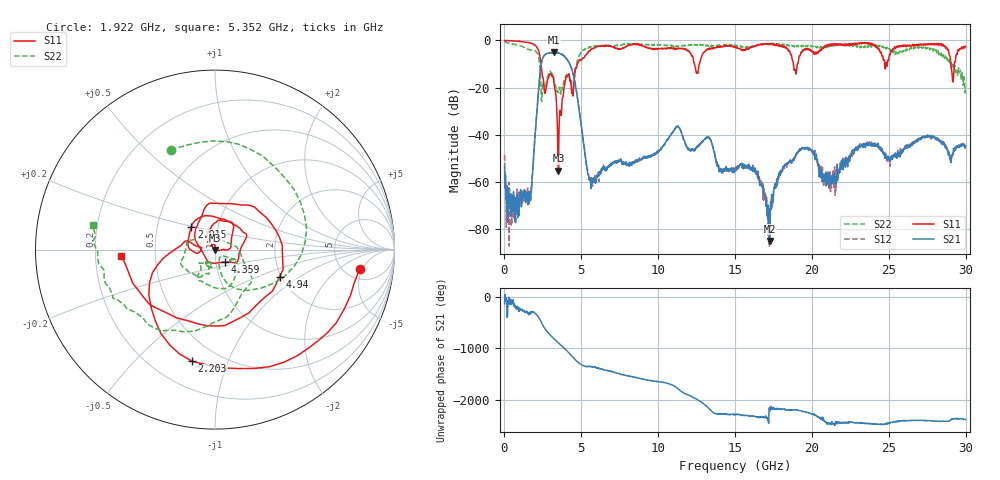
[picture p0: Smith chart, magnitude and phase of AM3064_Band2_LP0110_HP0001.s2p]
# Hz S DB R 50.0
!freq dBS11 angS11 dBS21 angS21 dBS12 angS12 dBS22 angS22
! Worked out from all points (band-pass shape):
!   1600 points, 10 MHz to 29.98 GHz, reference 50 ohm
!   highest |S21| = -5.00 dB at 3.234 GHz (marker M1); lowest = -84.9 dB at 17.27 GHz (marker M2)
!   |S21| within 3 dB of the highest: 2.462 GHz to 4.067 GHz (1.605 GHz wide, 49.2 % of centre)
!   lowest |S11| = -55.2 dB at 3.515 GHz (marker M3), VSWR 1.00, Z = 49.9 - j0.162 ohm
!   |S11| at or under -10 dB: 2.377 GHz to 4.741 GHz (2.364 GHz wide, 66.4 % of centre); 12.36 GHz to 12.67 GHz (317 MHz wide, 2.53 % of centre); 18.8 GHz to 19.05 GHz (253.7 MHz wide, 1.34 % of centre)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
!   |S22| runs from -25.8 to -0.2 dB; largest |S21 - S12| = 0.024
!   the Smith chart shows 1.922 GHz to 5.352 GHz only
!   S11 on the Smith chart (normalised r, x): 1.922 GHz: 6.80, -4.40; 2.203 GHz: 0.36, -0.75; 2.915 GHz: 0.74, +0.19; 4.359 GHz: 1.11, -0.15; 4.94 GHz: 1.96, -0.70; 5.352 GHz: 0.31, -0.03
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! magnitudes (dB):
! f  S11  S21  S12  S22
! 10 MHz  0.0  -53.6  -48.5  -0.2
! 591.1 MHz  -0.2  -64.1  -71.0  -1.6
! 1.622 GHz  -1.0  -66.6  -65.5  -4.0
! 1.922 GHz  -1.8  -46.8  -46.7  -4.3
! 2.203 GHz  -3.9  -22.2  -22.2  -6.3
! 2.522 GHz  -16.3  -7.1  -7.1  -17.4
! 2.915 GHz  -14.8  -5.3  -5.3  -13.4
! 3.234 GHz  -18.7  -5.0  -5.2  -18.0
! 3.515 GHz  -55.2  -5.3  -5.3  -21.9
! 4.359 GHz  -21.0  -11.7  -11.7  -20.0
! 4.94 GHz  -8.2  -33.2  -33.2  -5.3
! 5.015 GHz  -8.3  -36.7  -36.8  -5.1
! 5.352 GHz  -5.6  -53.2  -53.0  -3.2
! 10 GHz  -3.5  -47.0  -47.2  -1.9
! 11.27 GHz  -3.5  -36.5  -36.3  -2.6
! 15 GHz  -2.7  -55.0  -55.1  -2.1
! 17.27 GHz  -1.4  -84.9  -73.8  -1.3
! 18.25 GHz  -3.2  -53.0  -53.0  -1.8
! 19.99 GHz  -4.4  -46.6  -47.3  -2.3
! 21.25 GHz  -1.5  -59.0  -59.6  -2.5
! 25 GHz  -8.0  -49.8  -49.9  -3.2
! 29.98 GHz  -2.5  -44.8  -45.8  -20.2
